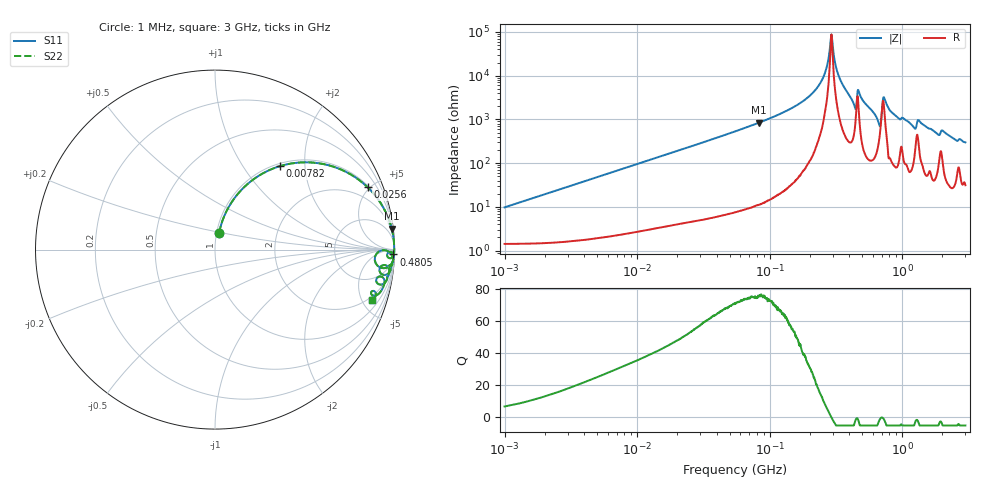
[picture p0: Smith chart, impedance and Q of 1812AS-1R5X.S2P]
!s-Parameter Generated by FASTRON Sdn. Bhd.
!FASTRON P/N : 1812AS-1R5X
!Keysight Technologies,E4991B,MY54100416,A.01.15
!Date created: Fri Oct 13 15:30:31 2023
!Version  : Rev00 Fri Oct 13 15:30:31 2023
!Data & Calibration Information:
!Freq	S11	S21	S12	S22
!PortZ  Port1:50+j0  Port2:50+j0
!When reading, reference impedance value at option line is always used.
! Remarks : This data is being provided solely for informational purposes.
# Hz S dB R 50
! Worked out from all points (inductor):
!   1601 points, 1 MHz to 3 GHz, reference 50 ohm
!   read as one part in series: L = 1.54 uH near 1.041 MHz
!   highest Q = 75.3 at 83.39 MHz (marker M1), where L = 1.61 uH
!   self-resonance near 291.3 MHz
!   S11 on the Smith chart (normalised r, x): 1 MHz: 1.03, +0.19; 7.82 MHz: 1.05, +1.49; 25.6 MHz: 1.09, +4.85; 480.5 MHz: 14, -71; 3 GHz: 1.63, -5.93
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1000000  -20.37 76.2  -0.16 -5.4  -0.16 -5.4  -20.37 76.2
3804036  -9.42 67.5  -0.68 -19.7  -0.68 -19.7  -9.42 67.5
7819618  -4.59 52.1  -2.05 -36.1  -2.05 -36.1  -4.59 52.1
1.447069e7  -1.95 35.6  -4.70 -53.0  -4.70 -53.0  -1.95 35.6
2.559965e7  -0.74 22.2  -8.44 -66.7  -8.44 -66.7  -0.74 22.2
5.477226e7  -0.17 10.6  -14.67 -78.5  -14.67 -78.5  -0.17 10.6
8.338914e7  -0.07 6.7  -18.62 -82.5  -18.62 -82.5  -0.07 6.7
2.083556e8  -0.01 1.5  -31.74 -86.5  -31.74 -86.5  -0.01 1.5
2.558035e8  -0.01 0.6  -39.77 -83.6  -39.77 -83.6  -0.01 0.6
2.92808e8  -0.01 -0.0  -58.86 2.7  -58.86 2.7  -0.01 -0.0
3.252521e8  -0.01 -0.5  -41.43 80.8  -41.43 80.8  -0.01 -0.5
3.631036e8  -0.01 -1.0  -34.95 84.0  -34.95 84.0  -0.01 -1.0
4.347762e8  -0.10 -2.6  -26.61 74.1  -26.61 74.1  -0.10 -2.6
4.805402e8  -0.05 -1.6  -31.20 78.1  -31.20 78.1  -0.05 -1.6
6.652545e8  -0.41 -6.2  -18.78 63.3  -18.78 63.3  -0.41 -6.2
7.316083e8  -0.16 -1.5  -30.04 54.7  -30.04 54.7  -0.16 -1.5
7.925923e8  -0.05 -3.2  -24.91 82.5  -24.91 82.5  -0.05 -3.2
1.218836e9  -0.28 -8.2  -16.82 73.0  -16.82 73.0  -0.28 -8.2
1.347129e9  -0.24 -5.9  -19.54 72.1  -19.54 72.1  -0.24 -5.9
1.837163e9  -0.41 -11.6  -13.85 71.3  -13.85 71.3  -0.41 -11.6
2.03054e9  -0.39 -9.9  -15.17 70.5  -15.17 70.5  -0.39 -9.9
3e9  -0.73 -17.8  -10.22 66.1  -10.22 66.1  -0.73 -17.8
